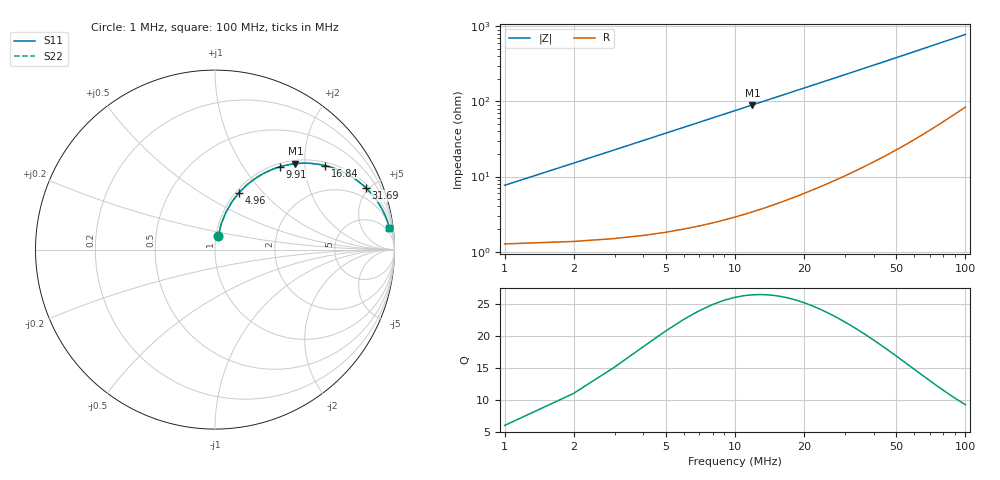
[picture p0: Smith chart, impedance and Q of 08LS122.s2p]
# MHz S MA R 50
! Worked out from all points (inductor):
!   101 points, 1 MHz to 100 MHz, reference 50 ohm
!   read as one part in series: L = 1.2 uH near 1 MHz
!   highest Q = 26.5 at 11.89 MHz (marker M1), where L = 1.2 uH
!   S11 on the Smith chart (normalised r, x): 1 MHz: 1.03, +0.15; 4.96 MHz: 1.04, +0.75; 9.91 MHz: 1.06, +1.49; 16.84 MHz: 1.10, +2.54; 31.69 MHz: 1.22, +4.80; 100 MHz: 3, +15
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1  0.07529 76.2  0.9848 -4.3  0.9848 -4.3  0.07529 76.2
1.99  0.147 76.4  0.9759 -8.4  0.9759 -8.4  0.147 76.4
2.98  0.2166 73.7  0.962 -12.5  0.962 -12.5  0.2166 73.7
3.97  0.2829 70.5  0.9438 -16.4  0.9438 -16.4  0.2829 70.5
4.96  0.3452 67.1  0.922 -20.2  0.922 -20.2  0.3452 67.1
6.94  0.4562 60.5  0.8711 -27.1  0.8711 -27.1  0.4562 60.5
7.93  0.5047 57.4  0.8433 -30.3  0.8433 -30.3  0.5047 57.4
9.91  0.5882 51.8  0.7865 -36.0  0.7865 -36.0  0.5882 51.8
11.89  0.6557 46.9  0.7307 -40.9  0.7307 -40.9  0.6557 46.9
13.87  0.71 42.6  0.678 -45.2  0.678 -45.2  0.71 42.6
16.84  0.7719 37.3  0.6068 -50.5  0.6068 -50.5  0.7719 37.3
17.83  0.7885 35.8  0.5853 -52.0  0.5853 -52.0  0.7885 35.8
20.8  0.829 31.8  0.5272 -55.9  0.5272 -55.9  0.829 31.8
23.77  0.859 28.5  0.4777 -59.1  0.4777 -59.1  0.859 28.5
27.73  0.888 25.0  0.4228 -62.5  0.4228 -62.5  0.888 25.0
31.69  0.9086 22.2  0.3781 -65.2  0.3781 -65.2  0.9086 22.2
34.66  0.9202 20.4  0.3498 -66.8  0.3498 -66.8  0.9202 20.4
41.59  0.9394 17.2  0.2968 -69.7  0.2968 -69.7  0.9394 17.2
50.5  0.9543 14.3  0.2474 -72.3  0.2474 -72.3  0.9543 14.3
67.33  0.9686 10.7  0.1869 -75.0  0.1869 -75.0  0.9686 10.7
84.16  0.9753 8.6  0.1496 -76.2  0.1496 -76.2  0.9753 8.6
100  0.9786 7.2  0.1256 -76.6  0.1256 -76.6  0.9786 7.2
